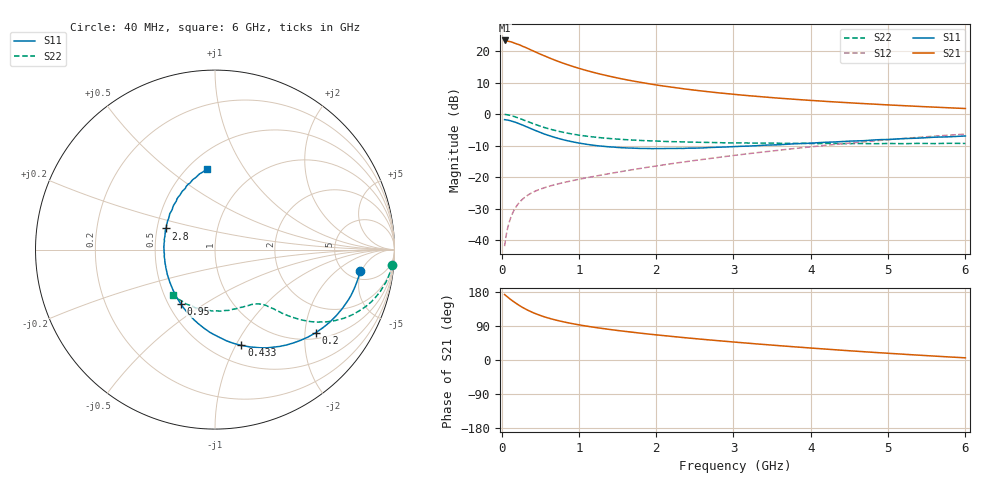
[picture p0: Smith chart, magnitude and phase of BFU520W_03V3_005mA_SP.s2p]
! Filename:  P:\Prog\Test\Noise\ATS_data\Testdata_Net\Run2\BFU520W_APM2013_06_A05_03p3V_005mA_SP_CM01_D.s2p
! Date/Time: Tue 26/Mar/2013 18:01:38
! BFU520W_APM2013_06_A05_03p3V_1to20mA_SP_CM01_Bias4_R.s2p
! MDIF S-parameter v. bias file
! BFU520W_APM2013_06_A05_03p3V_1to20mA_SP_CM01
! Date/time Tue Mar 19 16:47:37 2013
! VAR V_out= 3.3000
! VAR I_out= 4.9950
! VAR V_in= 0.8332
! VAR I_in= 0.0571
! Device data file deembeded for feedlines and parallel
! Original file: \Run2\BFU520W_APM2013_06_A05_03p3V_005mA_SP_CM01_R.s2p
! Feed-files: PR019V01_070313_Feed1.s2p, PR019V01_070313_Feed2.s2p
! Parallel-file: PR019V01_070313_Par.s2p
# MHz S MA R 50
!  Freq-MHz  S11-mag  S11-arg  S21-mag  S21-arg  S12-mag  S12-arg  S22-mag  S22-arg
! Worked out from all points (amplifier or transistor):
!   98 points, 40 MHz to 6 GHz, reference 50 ohm
!   highest |S21| = 23.4 dB at 40 MHz (marker M1)
!   |S21| within 3 dB of that: start of sweep to 379.2 MHz
!   unconditionally stable (mu >= 1): 1.769 GHz to 3.067 GHz
!   at 300 MHz: K = 0.33, MSG = 23.9 dB, |S12| = -26.4 dB
!   at 1.6 GHz: K = 0.98, MSG = 14.5 dB, |S12| = -18.0 dB
!   at 6 GHz: K = 0.87, MSG = 4.1 dB, |S12| = -6.3 dB
!   S11 on the Smith chart (normalised r, x): 40 MHz: 6.50, -4.68; 200 MHz: 1.15, -2.27; 433 MHz: 0.69, -1.05; 950 MHz: 0.58, -0.40; 2.8 GHz: 0.56, +0.14; 6 GHz: 0.62, +0.69
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40  0.8169 -8.4  14.79 172.8  0.008008 84.9  0.9901 -4.9
50  0.815 -10.5  14.79 171.0  0.009937 84.3  0.9881 -6.0
120  0.7817 -24.8  14.11 159.5  0.02286 77.0  0.9502 -14.2
160  0.7564 -32.4  13.56 153.5  0.02956 73.2  0.9202 -18.3
200  0.7275 -39.6  12.98 148.0  0.03547 70.0  0.8847 -22.0
240  0.695 -46.6  12.48 142.6  0.04081 67.3  0.8493 -25.2
320  0.6321 -59.4  11.33 133.4  0.04978 62.9  0.7777 -30.5
380  0.5887 -67.7  10.46 127.5  0.05531 60.5  0.7283 -33.6
433  0.5528 -74.6  9.783 122.9  0.0597 59.0  0.6901 -35.8
550  0.4847 -88.2  8.472 114.2  0.06751 56.7  0.6158 -39.3
650  0.4421 -98.0  7.53 108.2  0.07359 55.9  0.5688 -41.3
800  0.3916 -111.0  6.421 100.8  0.08178 55.6  0.5148 -43.5
950  0.3571 -122.3  5.583 94.7  0.08964 56.0  0.4755 -44.9
1050  0.3398 -129.2  5.127 91.1  0.09484 56.5  0.4555 -45.8
1250  0.314 -141.7  4.406 84.8  0.1056 57.5  0.426 -47.3
1500  0.2961 -155.0  3.753 77.9  0.1197 58.6  0.4015 -49.6
2050  0.2837 -178.7  2.848 65.3  0.1533 60.1  0.3714 -55.2
2800  0.2983 156.7  2.184 51.0  0.2052 59.9  0.3527 -66.0
3100  0.3087 148.6  2.012 45.8  0.2282 59.1  0.3497 -70.7
4100  0.3527 127.0  1.624 30.1  0.3113 54.3  0.3408 -89.4
5200  0.4087 107.7  1.363 15.2  0.4107 46.0  0.3396 -113.2
6000  0.4505 95.8  1.228 5.7  0.4823 38.6  0.3424 -132.8
